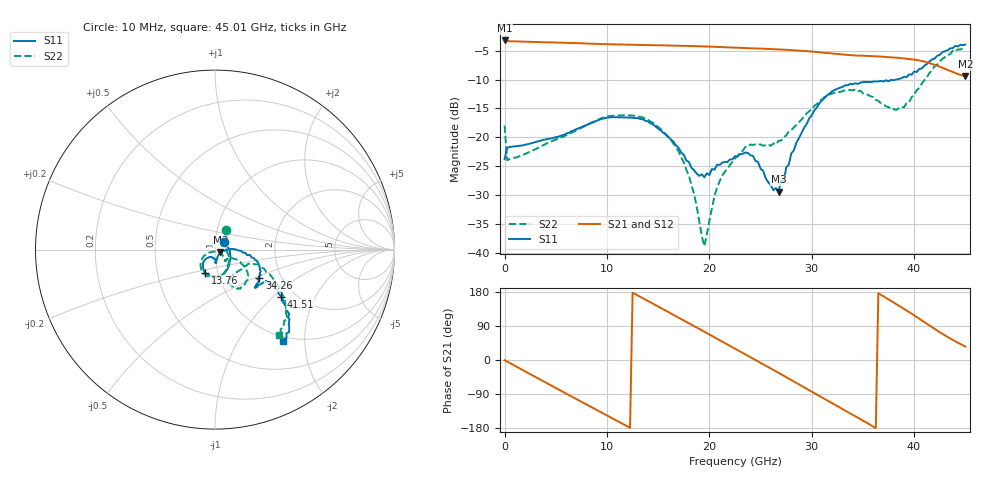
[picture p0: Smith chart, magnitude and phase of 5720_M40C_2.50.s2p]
! Device:  ADRF5720
! Description: 0.5dB LSB GaAs MMIC 6-bit Digital Attenuator
! Frequency:  0.000009 -  40 GHz
! Ports:
!	RF1	= Port 1
!	RF2	= Port 2
! Vdd:  3.3 Volt
! Vss:  -3.3 Volt
! Control:  0/3.3 Volt
! State:  2.50 dB attenuation
! Data:  The device was measured using G-S-G Probes on a matrix board.
!  Data was collected using an calibrated 4 port network analyzer.
!  The reference plane for this measurement is at the launchers.
! Note:  Analog Devices supplies this data as a sample of measured data
!  for this product.  Your particular data for this product may vary.
!  Data was taken at -40 degrees C.
!  Analog Devices reserves the right to change this data at anytime.
# GHZ S DB R 45.0
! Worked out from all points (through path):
!   181 points, 10 MHz to 45.01 GHz, reference 45 ohm
!   highest |S21| = -3.22 dB at 10 MHz (marker M1); lowest = -9.4 dB at 45.01 GHz (marker M2)
!   group delay of S21, straight-line fit = 42 ps
!   lowest |S11| = -29.4 dB at 26.76 GHz (marker M3), VSWR 1.07, Z = 47.7 - j1.52 ohm
!   |S11| at or under -10 dB: start of sweep to 38.24 GHz
!   |S22| runs from -38.9 to -4.5 dB; largest |S21 - S12| = 0.0025
!   S11 on the Smith chart (normalised r, x): 10 MHz: 1.10, +0.09; 13.76 GHz: 0.87, -0.23; 34.26 GHz: 1.54, -0.54; 41.51 GHz: 1.71, -1.13; 45.01 GHz: 0.92, -1.58
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0.01  -23.79 41.2  -3.22 -0.9  -3.24 -0.9  -17.99 62.3
0.26  -21.81 0.9  -3.34 -4.1  -3.36 -4.1  -23.98 1.6
2.01  -21.31 -14.2  -3.43 -30.0  -3.45 -30.1  -22.90 -14.3
4.26  -20.27 -26.3  -3.54 -63.0  -3.56 -63.0  -20.94 -28.0
7.76  -18.04 -54.8  -3.73 -113.9  -3.75 -113.9  -18.12 -57.7
10.76  -16.53 -82.0  -3.90 -157.2  -3.92 -157.3  -16.26 -87.0
13.76  -17.14 -113.2  -4.02 159.4  -4.04 159.3  -16.80 -118.0
15.26  -18.81 -126.0  -4.06 137.5  -4.07 137.4  -18.59 -133.3
18.01  -24.31 -130.5  -4.17 97.0  -4.19 96.9  -26.66 -155.1
19.51  -26.94 -108.1  -4.26 74.7  -4.28 74.6  -38.88 -87.0
20.76  -24.76 -87.1  -4.34 56.1  -4.36 56.1  -28.72 -33.8
22.76  -23.34 -87.6  -4.48 26.4  -4.50 26.3  -23.22 -42.5
24.26  -23.21 -85.6  -4.59 4.0  -4.61 3.9  -21.34 -48.2
26.76  -29.44 -28.1  -4.78 -33.8  -4.80 -34.0  -20.60 -32.2
28.01  -22.80 -0.3  -4.89 -52.9  -4.91 -53.0  -18.73 -26.7
30.26  -15.37 -6.0  -5.18 -87.7  -5.20 -87.9  -14.55 -30.0
32.01  -12.01 -17.1  -5.48 -114.4  -5.50 -114.5  -12.42 -40.2
34.26  -10.64 -32.8  -5.83 -148.4  -5.85 -148.5  -11.70 -57.1
37.76  -10.04 -41.2  -6.15 155.8  -6.17 155.6  -15.20 -58.6
39.51  -9.10 -31.9  -6.45 126.6  -6.47 126.4  -14.00 -23.6
41.51  -6.87 -35.3  -7.16 90.6  -7.18 90.4  -8.83 -26.6
45.01  -3.93 -53.4  -9.42 35.3  -9.45 35.1  -4.51 -53.2
